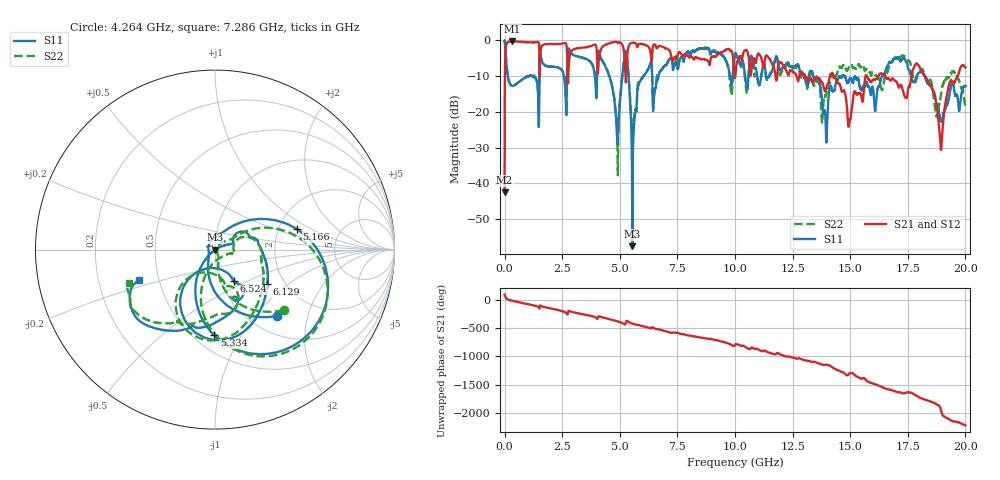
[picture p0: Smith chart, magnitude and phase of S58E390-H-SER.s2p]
!{S58E390}
!Johanson Technology Inc.
!www.johansontechnology.com
!Test Board Conditions:
!Substrate Type  RO4350B
!Substrate Thickness  60 mil
!Substrate Dk  3.66
!TL Type: GCPW
!TL Trace Width  115 mil
!TL Gap  52 mil
!Electrode orientation  Horizontal
!DUT TOPOLOGY	SERIES
!Mounting Pad LxW  55x428 mil
! Created Wed Apr 14 11:45:53 2021
# mhz S ma R 50
! 2 Port Network Data from SP1.SP block
! freq  magS11  angS11  magS21  angS21  magS12  angS12  magS22  angS22
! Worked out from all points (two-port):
!   20001 points, 300 kHz to 20 GHz, reference 50 ohm
!   highest |S21| = -0.26 dB at 335.3 MHz (marker M1); lowest = -42.4 dB at 300 kHz (marker M2)
!   |S21| within 3 dB of the highest: 37.93 MHz to 1.509 GHz (1.471 GHz wide, 190 % of centre); 1.559 GHz to 2.71 GHz (1.152 GHz wide, 53.9 % of centre)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
!   lowest |S11| = -57.5 dB at 5.543 GHz (marker M3), VSWR 1.00, Z = 50 - j0.13 ohm
!   |S11| at or under -10 dB: 13.39 GHz to 14.54 GHz (1.145 GHz wide, 8.2 % of centre); 14.74 GHz to 16.38 GHz (1.641 GHz wide, 10.5 % of centre); 18.21 GHz to end of sweep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
!   |S22| runs from -37.7 to 0.0 dB; largest |S21 - S12| = 0.011
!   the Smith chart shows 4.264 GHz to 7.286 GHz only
!   S11 on the Smith chart (normalised r, x): 4.264 GHz: 1.32, -1.30; 5.166 GHz: 2.51, +0.74; 5.334 GHz: 0.63, -0.77; 6.129 GHz: 1.63, -0.72; 6.524 GHz: 1.15, -0.42; 7.286 GHz: 0.39, -0.17
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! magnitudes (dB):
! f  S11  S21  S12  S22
! 300 kHz  0.0  -42.4  -42.4  0.0
! 108.3 MHz  -8.5  -0.7  -0.7  -8.5
! 335.3 MHz  -12.7  -0.3  -0.3  -12.7
! 3.334 GHz  -4.8  -2.1  -2.1  -4.7
! 4.264 GHz  -5.9  -1.7  -1.7  -5.9
! 4.89 GHz  -28.0  -0.5  -0.5  -26.7
! 5.166 GHz  -6.6  -2.5  -2.5  -6.4
! 5.334 GHz  -6.4  -3.4  -3.4  -6.2
! 5.543 GHz  -57.5  -0.7  -0.6  -25.2
! 6.129 GHz  -9.1  -1.3  -1.3  -9.1
! 6.524 GHz  -13.7  -1.1  -1.2  -13.5
! 6.667 GHz  -10.6  -1.8  -1.8  -8.8
! 7.286 GHz  -6.8  -5.9  -5.8  -5.8
! 10 GHz  -3.7  -10.5  -10.5  -3.9
! 13.33 GHz  -8.6  -11.4  -11.3  -10.3
! 13.92 GHz  -21.0  -14.2  -14.1  -15.7
! 14.97 GHz  -11.0  -22.7  -22.7  -7.0
! 16.1 GHz  -19.3  -10.8  -10.8  -9.8
! 16.67 GHz  -6.4  -10.6  -10.6  -7.8
! 17.95 GHz  -9.2  -6.9  -6.8  -9.6
! 18.94 GHz  -22.4  -30.4  -30.2  -15.2
! 20 GHz  -12.7  -7.5  -7.5  -18.8
